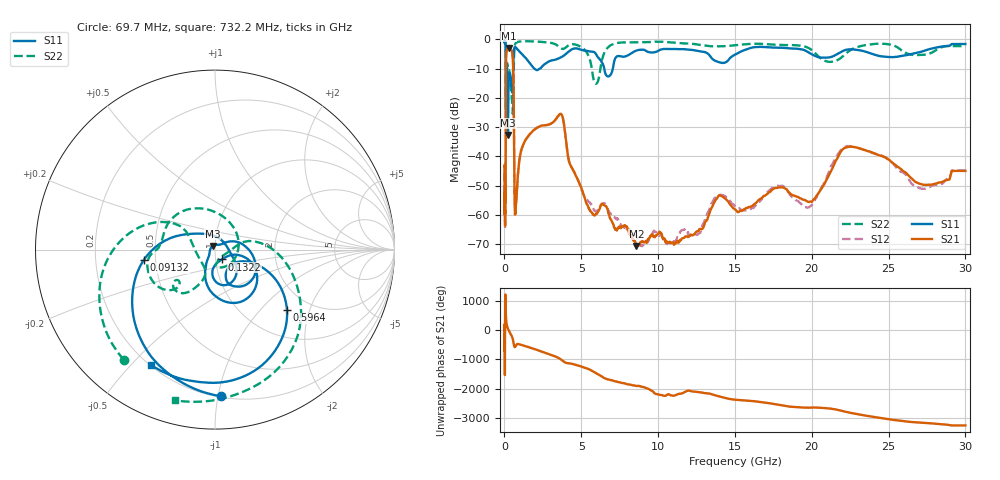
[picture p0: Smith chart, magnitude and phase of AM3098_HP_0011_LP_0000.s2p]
! Date/Time: Thu, Feb 28, 2019 8:33 AM
! Network Analyzer: Agilent Technologies E8364B Rev: A.07.50.67
! Sweep from 0.010 to 30.000 GHz, 1601 Points, Sweep Type: LOG
! Power Supply: 5.022 V, 0.002 A
# Hz S DB R 50
!freq MagS11 AngS11 MagS21 AngS21 MagS12 AngS12 MagS22 AngS22
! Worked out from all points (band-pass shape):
!   1601 points, 10 MHz to 30 GHz, reference 50 ohm
!   highest |S21| = -2.95 dB at 266.5 MHz (marker M1); lowest = -70.7 dB at 8.587 GHz (marker M2)
!   |S21| within 3 dB of the highest: 107.6 MHz to 533.9 MHz (426.3 MHz wide, 133 % of centre)
!   lowest |S11| = -32.7 dB at 229.3 MHz (marker M3), VSWR 1.05, Z = 48.8 + j1.94 ohm
!   |S11| at or under -10 dB: 175.9 MHz to 562.1 MHz (386.2 MHz wide, 105 % of centre); 1.955 GHz to 2.284 GHz (329.2 MHz wide, 15.5 % of centre); 6.496 GHz to 7.051 GHz (554.5 MHz wide, 8.19 % of centre)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
!   |S22| runs from -25.5 to -0.5 dB; largest |S21 - S12| = 0.01
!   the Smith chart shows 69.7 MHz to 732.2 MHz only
!   S11 on the Smith chart (normalised r, x): 69.7 MHz: 0.21, -1.02; 91.32 MHz: 0.43, -0.06; 132.2 MHz: 1.07, -0.12; 596.4 MHz: 1.53, -1.43; 732.2 MHz: 0.20, -0.57
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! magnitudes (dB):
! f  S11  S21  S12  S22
! 10 MHz  -0.3  -43.2  -45.5  -0.5
! 38.04 MHz  -0.5  -61.8  -59.1  -0.8
! 69.7 MHz  -1.8  -55.2  -53.6  -2.0
! 91.32 MHz  -7.9  -19.9  -19.8  -9.5
! 100.9 MHz  -23.9  -8.0  -8.0  -17.6
! 132.2 MHz  -23.5  -3.9  -3.9  -11.5
! 144.7 MHz  -14.4  -3.6  -3.5  -10.4
! 187.7 MHz  -11.5  -3.4  -3.4  -8.3
! 229.3 MHz  -32.7  -3.0  -3.0  -10.0
! 266.5 MHz  -15.3  -3.0  -2.9  -10.5
! 550.5 MHz  -12.0  -7.2  -7.2  -25.3
! 596.4 MHz  -5.6  -17.1  -17.0  -10.9
! 665.8 MHz  -2.6  -56.2  -55.5  -2.3
! 732.2 MHz  -2.7  -57.9  -57.1  -1.2
! 2.084 GHz  -10.5  -30.3  -30.3  -0.7
! 3.686 GHz  -6.1  -25.5  -25.5  -3.0
! 5.959 GHz  -5.0  -59.5  -58.7  -15.1
! 7.926 GHz  -5.7  -64.0  -65.3  -1.0
! 8.587 GHz  -3.8  -70.7  -67.3  -1.0
! 19.7 GHz  -4.2  -55.4  -57.5  -2.7
! 22.67 GHz  -3.4  -36.7  -36.7  -3.2
! 30 GHz  -1.6  -45.0  -44.8  -2.3
